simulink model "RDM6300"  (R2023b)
settings: Solver=FixedStepAuto  StartTime=0.0  StopTime=inf  RelTol=1e-3  EnableMultiTasking=on
libraries: arduinolib x5

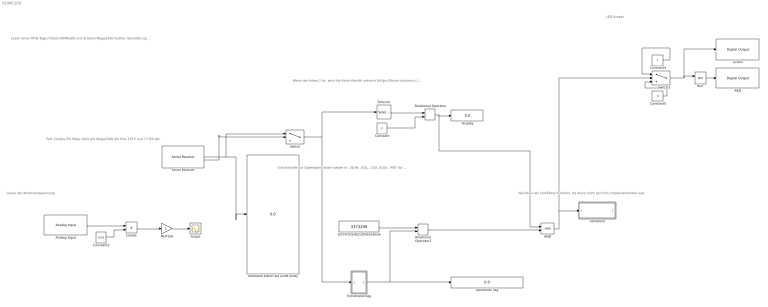
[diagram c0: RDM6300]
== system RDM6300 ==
  note: Port 2(siehe Pin Map) stellt am Mega2560 die Pins 16TX und 17 RX dar.
  note: Schnittstelle zur Datenbank leider weder in: .JSON, .SQL, .CSV,.XLSX, .MAT für Strings umsetzbar. Darum kann der Tag nicht sinnvoll mit einem Namen verglichen werden. Es können zwar Tags und eine ID dazu in einer externen Datei gespeichert werden, doch müssen die Namen als String immer fest im Matlab modell eingetragen sein. Das unter solchen bedingungen getrennt in einer "Datenbank" und einer Datei wie diesem modell zu halten ist unrealistisch und aufwändig
  note: Nachbau der SendTone Funktion, da diese nicht per fcn() implementierbar war.
  note: Lesen der Antennenspannung
  note: LED-Ampel
  note: Wenn der Index 2 ist, wird die Karte Korrekt erkannt [https://forum.arduino.cc/t/rdm6300-reading-format/1072597]
  note: Lesen eines RFID Tags mittels RDM6300 und Arduino Mega2560 Author: Benedikt Lipinski Studiengang: Business and Systems Engineering Hochschule: Hamm-Lippstadt Datum: 28.04.2024 Version 1.0 Matlab/Simulink: 2023b Packages: Hardware Support for Arduino
  AND : Logic  IconShape=distinctive  AllPortsSameDT=off  OutDataTypeStr=boolean
  Analog Input : arduinolib/Analog Input  Commented=on  pinNumber=0  ReadResultsOnly=off  ConversionTriggerSource=Software  ExternalTriggerType=uint32( 0 )  OutputDataType=uint16  EnableConversionCompleteNotify=off  EnableOuputStatus=off  SampleTime=-1  blockPlatform=arduino
  Constant : Constant  Value=2
  Constant2 : Constant  Commented=on  Value=1023
  Constant4 : Constant  Commented=on
  Constant5 : Constant  Commented=on  Value=0
  Display : Display
  Divide : Product  Commented=on  Inputs=*/
  ExtrahierenTag : Subsystem
  Gelesene Daten als uint8 Array : Display
  Gelesener Tag : Display
  Green : arduinolib/Digital Output  Commented=on  pinNumber=52  Direction=output  blockPlatform=arduino
  Multiply : Gain  Commented=on  Gain=5
  NOT : Logic  Commented=on  Operator=NOT  IconShape=distinctive  AllPortsSameDT=off  OutDataTypeStr=boolean
  RED : arduinolib/Digital Output  Commented=on  pinNumber=51  Direction=output  blockPlatform=arduino
  Relational Operator : RelationalOperator  Operator===  OutDataTypeStr=boolean  RndMeth=Simplest
  Relational Operator1 : RelationalOperator  Operator===  OutDataTypeStr=boolean  RndMeth=Simplest
  SchnittstelleZurDatenbank : Constant  Value=3373299
  Scope : Scope
  Selector : Selector  InputPortWidth=14  IndexOptions=Starting index (dialog)  Indices=1  OutputSizes=1
  SendTone : Subsystem
  Serial Receive : arduinolib/Serial Receive  isARMArch=off  portNumber=2  DataType=uint8  Datalength=14  SampleTime=0.1  showOutStatus=on  blockPlatform=arduino
  Switch : Switch  Criteria=u2 > Threshold
  Switch3 : Switch  Commented=on  Criteria=u2 > Threshold
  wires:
  Constant/1 -> Relational Operator/2
  Selector/1 -> Relational Operator/1
  Relational Operator/1 -> AND/1, Display/1
  ExtrahierenTag/1(y) -> Relational Operator1/2, Gelesener Tag/1
  Constant4/1 -> Switch3/1
  Constant5/1 -> Switch3/3
  NOT/1 -> RED/1
  Switch3/1 -> Green/1, NOT/1
  Relational Operator1/1 -> AND/2
  AND/1 -> Switch3/2, SendTone/1(In1)
  Switch/1 -> ExtrahierenTag/1(In1), Selector/1
  Serial Receive/1 -> Switch/1, Gelesene Daten als uint8 Array/1
  Serial Receive/2 -> Switch/2
  SchnittstelleZurDatenbank/1 -> Relational Operator1/1
  Analog Input/1 -> Divide/1
  Constant2/1 -> Divide/2
  Divide/1 -> Multiply/1
  Multiply/1 -> Scope/1

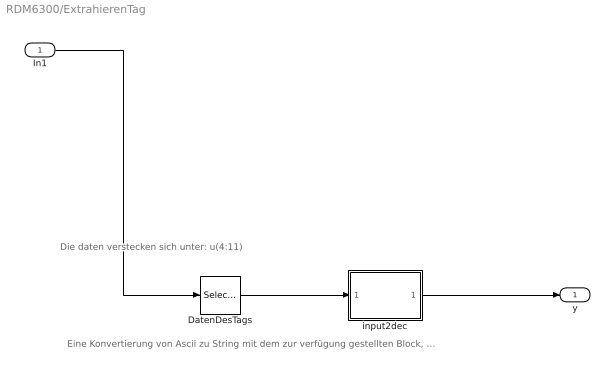
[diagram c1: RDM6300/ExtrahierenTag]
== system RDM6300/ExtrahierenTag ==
  note: Eine Konvertierung von Ascii zu String mit dem zur verfügung gestellten Block, konnte aufgrund eines BITROL fehlers in der Funktion nicht genutzt werden. Von einer Fehlersuche in schreibgeschützten und durch Matlab zur verfügugn gestellten Funktioen habe ich abgesehen. Alle Fehler in diesem Zusammenhang stehen als Screenshot zur verfügung
  note: Die daten verstecken sich unter: u(4:11)
  In1 : Inport
  DatenDesTags : Selector  InputPortWidth=14  IndexOptions=Index vector (dialog)  Indices=[4 5 6 7 8 9 10 11]  OutputSizes=1
  input2dec : MATLAB Function  TreatAsAtomicUnit=on
  y : Outport
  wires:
  In1/1 -> DatenDesTags/1
  DatenDesTags/1 -> input2dec/1(u)
  input2dec/1(y) -> y/1

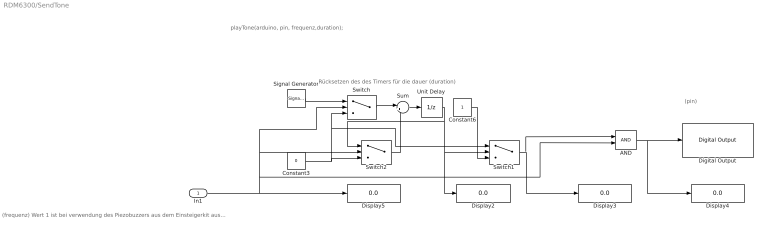
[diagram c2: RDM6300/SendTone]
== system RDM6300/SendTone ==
  note: (frequenz) Wert 1 ist bei verwendung des Piezobuzzers aus dem Einsteigerkit ausreichend aufmerksamkeitsfordernd
  note: (pin)
  note: playTone(arduino, pin, frequenz,duration);
  note: Rücksetzen des des Timers für die dauer (duration)
  In1 : Inport
  AND : Logic  IconShape=distinctive  AllPortsSameDT=off  OutDataTypeStr=boolean
  Constant3 : Constant  Value=0
  Constant6 : Constant
  Digital Output : arduinolib/Digital Output  pinNumber=53  Direction=output  blockPlatform=arduino
  Display{2..5} (4 alike) : Display
  Signal Generator : SignalGenerator  Frequency=0.1  Units=rad/sec
  Sum : Sum  Inputs=|++
  Switch : Switch  Criteria=u2 > Threshold
  Switch1 : Switch  Criteria=u2 > Threshold  Threshold=1
  Switch2 : Switch  Criteria=u2 > Threshold
  Unit Delay : UnitDelay  SampleTime=-1  HasFrameUpgradeWarning=on
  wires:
  Unit Delay/1 -> Switch2/1, Display2/1, Switch1/2
  Switch/1 -> Sum/1
  Constant3/1 -> Switch2/3, Switch1/1, Switch/3
  Constant6/1 -> Switch1/3
  AND/1 -> Display4/1, Digital Output/1
  Signal Generator/1 -> Switch/1
  Switch1/1 -> AND/1, Display3/1
  Sum/1 -> Unit Delay/1
  Switch2/1 -> Sum/2
  In1/1 -> Switch2/2, Switch/2, AND/2, Display5/1

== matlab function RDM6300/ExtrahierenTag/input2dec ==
% Die Daten aus dem Uint array repräsentieren einen ASCII wert. Der
% Ascii Wert wiederrum ergibt concatiniert einen Großen hex wert. im fall
% des benutzen tags '003378F3' Dieser Wert ergibt konvertiert die gesuchte zahl, unseren Tag.  
% Eine Simulink blockiert sich gerade bei der Verkettung und Umwandlung von
% strings oder dem entsprechend ganzen Char Arrays, weswegen an dieser
% stelle auf die verwendung von schleifen zurück gegriffen werden musst. 
function y = fcn(u)
    uint8Array = u
    decimalValue = uint32(0);
    for i = 1:8 % 8, weil 4 -11 
        % Addiere den aktuellen Wert zum Gesamtwert
        % Shift den aktuellen Wert auf die entsprechende Position
        decimalValue = decimalValue * 16 + hex2dec(char(uint8Array(i)));
    end
    y = decimalValue
end
